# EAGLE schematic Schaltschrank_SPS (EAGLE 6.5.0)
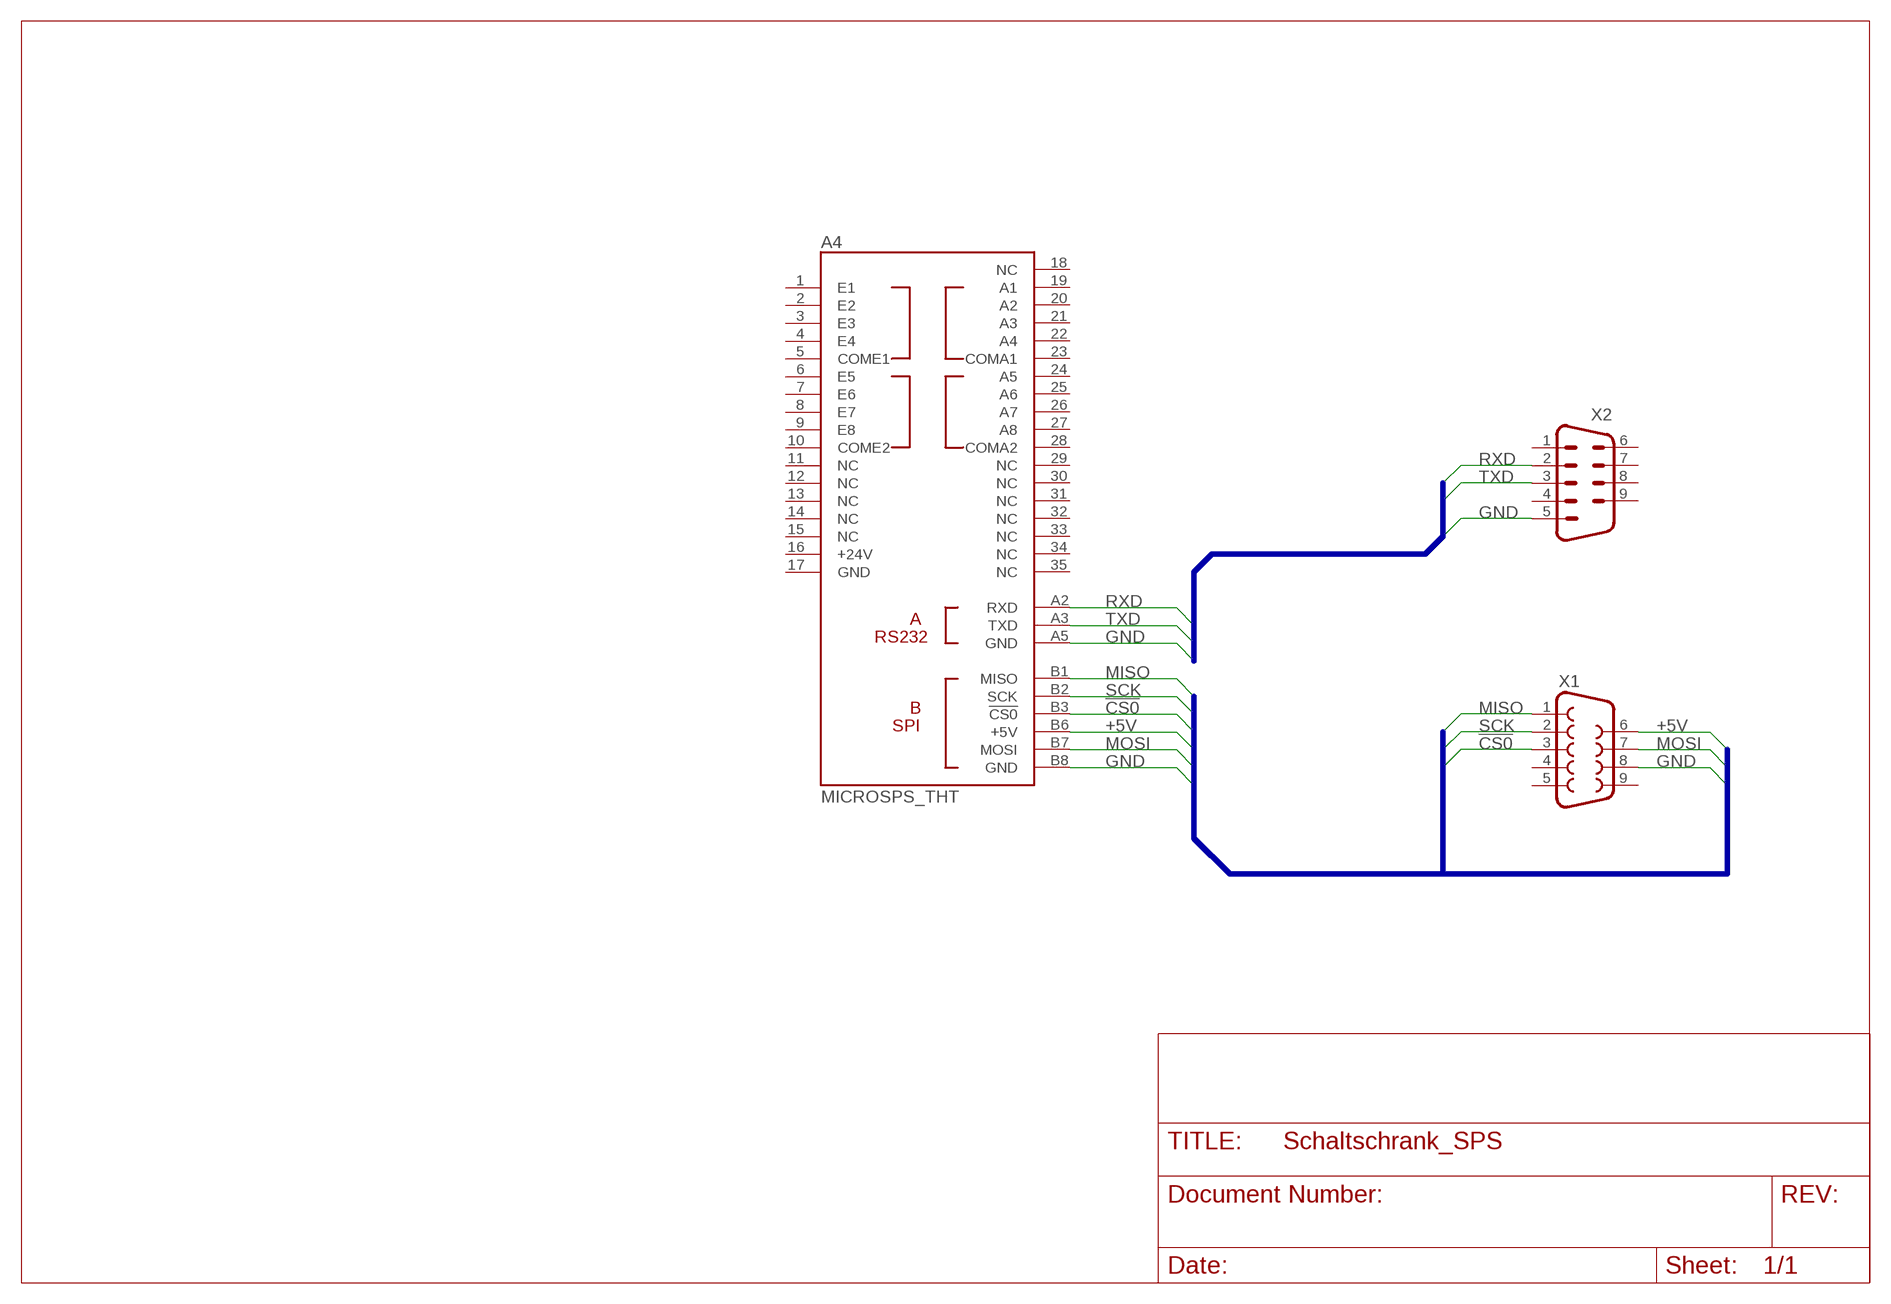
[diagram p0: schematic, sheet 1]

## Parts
A4  MICROSPS_THT  [MICROSPS]
X1  F09D  [F09D]
X2  M09D  [M09D]

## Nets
!CS0: A4.B3(!CS0) X1.3
+5V: A4.B6(+5V) X1.6
GND: A4.A5(GND) A4.B8(GND) X1.8 X2.5
MISO: A4.B1(MISO) X1.1
MOSI: A4.B7(MOSI) X1.7
RXD: A4.A2(RXD) X2.2
SCK: A4.B2(SCK) X1.2
TXD: A4.A3(TXD) X2.3
Unconnected: A4.1(E1) A4.2(E2) A4.3(E3) A4.4(E4) A4.5(COME1) A4.6(E5) A4.7(E6) A4.8(E7) A4.9(E8) A4.10(COME2) A4.11(NC) A4.12(NC) A4.13(NC) A4.14(NC) A4.15(NC) A4.16(+24V) A4.17(GND) A4.18(NC) A4.19(A1) A4.20(A2) A4.21(A3) A4.22(A4) A4.23(COMA1) A4.24(A5) A4.25(A6) A4.26(A7) A4.27(A8) A4.28(COMA2) A4.29(NC) A4.30(NC) A4.31(NC) A4.32(NC) A4.33(NC) A4.34(NC) A4.35(NC) X1.4 X1.5 X1.9 X2.1 X2.4 X2.6 X2.7 X2.8 X2.9

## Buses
MISO,SCK,!CS0,+5V,MOSI,GND
RXD,TXD,GND

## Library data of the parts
A4 = Brunner:MICROSPS_THT
X1 = con-subd:F09: SUB-D; OC_FARNELL: unknown; OC_NEWARK: unknown
X2 = con-subd:M09: SUB-D; OC_FARNELL: unknown; OC_NEWARK: unknown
